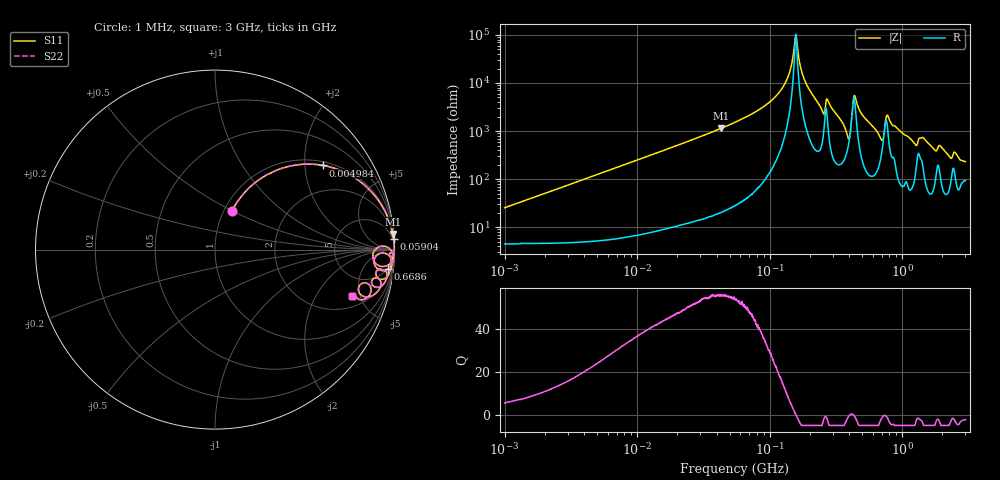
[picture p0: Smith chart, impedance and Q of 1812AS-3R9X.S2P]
!s-Parameter Generated by FASTRON Sdn. Bhd.
!FASTRON P/N : 1812AS-3R9X
!Keysight Technologies,E4991B,MY54100416,A.01.15
!Date created: Fri Oct 13 15:56:55 2023
!Version  : Rev00 Fri Oct 13 15:56:55 2023
!Data & Calibration Information:
!Freq	S11	S21	S12	S22
!PortZ  Port1:50+j0  Port2:50+j0
!When reading, reference impedance value at option line is always used.
! Remarks : This data is being provided solely for informational purposes.
# Hz S dB R 50
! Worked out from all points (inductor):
!   1601 points, 1 MHz to 3 GHz, reference 50 ohm
!   read as one part in series: L = 3.97 uH near 1.041 MHz
!   highest Q = 56.1 at 43.08 MHz (marker M1), where L = 4.21 uH
!   self-resonance near 157.4 MHz
!   S11 on the Smith chart (normalised r, x): 1 MHz: 1.09, +0.50; 4.984 MHz: 1.10, +2.48; 59.04 MHz: 2, +33; 668.6 MHz: 5, -16; 3 GHz: 2.84, -4.22
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1000000  -12.53 66.4  -0.62 -13.5  -0.62 -13.5  -12.53 66.4
3804036  -3.46 44.9  -3.01 -42.1  -3.01 -42.1  -3.46 44.9
4984223  -2.34 37.9  -4.23 -49.7  -4.23 -49.7  -2.34 37.9
1.447069e7  -0.37 15.4  -11.53 -73.3  -11.53 -73.3  -0.37 15.4
4.307715e7  -0.05 5.0  -21.18 -84.0  -21.18 -84.0  -0.05 5.0
5.477226e7  -0.03 3.8  -23.66 -85.2  -23.66 -85.2  -0.03 3.8
5.904167e7  -0.03 3.4  -24.49 -85.5  -24.49 -85.5  -0.03 3.4
1.201581e8  -0.01 0.8  -36.68 -85.9  -36.68 -85.9  -0.01 0.8
1.396205e8  -0.01 0.4  -43.56 -81.9  -43.56 -81.9  -0.01 0.4
1.574367e8  -0.01 0.0  -60.20 -5.9  -60.20 -5.9  -0.01 0.0
1.784169e8  -0.01 -0.4  -43.03 80.5  -43.03 80.5  -0.01 -0.4
2.083556e8  -0.01 -1.0  -35.49 84.0  -35.49 84.0  -0.01 -1.0
2.519921e8  -0.10 -2.2  -28.00 71.8  -28.00 71.8  -0.10 -2.2
2.771263e8  -0.05 -1.3  -32.32 74.3  -32.32 74.3  -0.05 -1.3
3.894533e8  -0.71 -5.7  -18.17 47.4  -18.17 47.4  -0.71 -5.7
4.435663e8  -0.10 -0.9  -34.03 52.5  -34.03 52.5  -0.10 -0.9
6.685918e8  -0.29 -6.5  -18.70 70.5  -18.70 70.5  -0.29 -6.5
7.064253e8  -0.89 -6.3  -16.90 44.0  -16.90 44.0  -0.89 -6.3
7.925923e8  -0.16 -2.9  -25.47 67.9  -25.47 67.9  -0.16 -2.9
1.243477e9  -0.42 -9.9  -15.11 69.4  -15.11 69.4  -0.42 -9.9
1.409185e9  -0.44 -7.1  -17.74 64.3  -17.74 64.3  -0.44 -7.1
3e9  -1.86 -18.7  -9.11 47.7  -9.11 47.7  -1.86 -18.7
